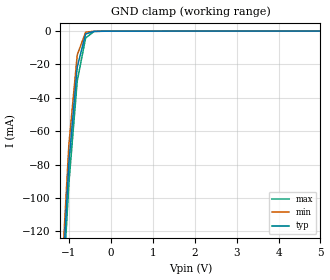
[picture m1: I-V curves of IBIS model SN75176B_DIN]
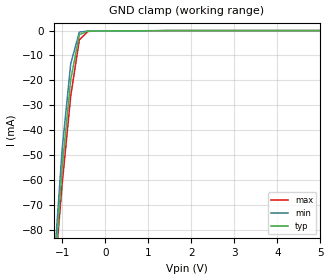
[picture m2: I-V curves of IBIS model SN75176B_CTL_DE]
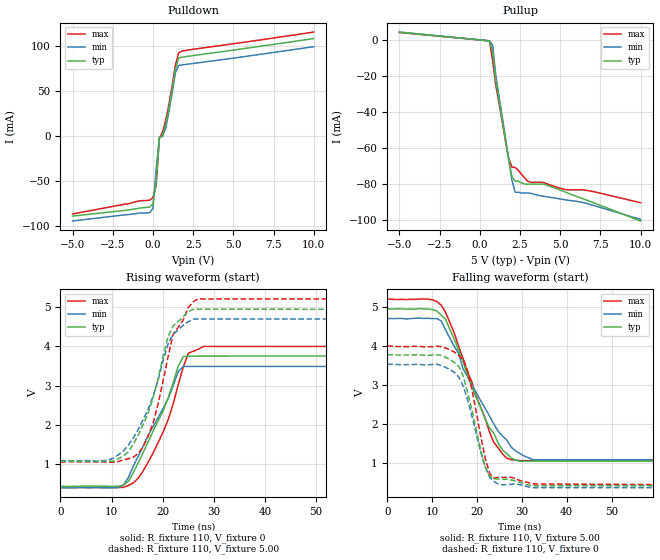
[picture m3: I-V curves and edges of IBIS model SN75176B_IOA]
|   TEXAS INSTRUMENTS INCORPORATED
|   Standard Linear and Logic Group
|   IBIS Model of SN75176
|   DIFFERENTIAL BUS TRANSCEIVERS
|   DIP 8-pin(P), SOL 8-pin(D), SOP 8-pin(PS)
[IBIS Ver]   3.1
[Comment char] |_char
[File Name]   sn75176b.ibs
[File Rev]   1.1
[Date]   Apr 26, 2004
[Source]   File originated at Texas Instruments, Inc
[Notes]   The following is a sample IBIS file for the SN75176B.
   - FILE REV HISTORY
   - 1.1 Release IBIS file on 04/29/04
   - All test data contained in this file are derived from
   actual measurement.
   - The measurement used P package.
   - We have data across voltage and temperature, but not across
   process.
[Disclaimer] Property of Texas Instruments Incorporated.  Unauthorized
   reproduction and/or distribution is strictly prohibited.
   This product is protected under copyright law.
   Created  2002, (C) Copyright  2002, Texas Instruments
   Incorporated, All Rights Reserved
   UNLESS THERE IS A SIGNED, WRITTEN AGREEMENT TO THE
   CONTRARY, TEXAS INSTRUMENTS (TI) IS PROVIDING THE IBIS
   MODELS  AND WITHOUT ANY WARRANTY, EXPRESSED OR
   IMPLIED.  TI assumes no liability for:
   1) the accuracy of the IBIS models provided to your
   company;
   2) the proper functioning of these IBIS Models in your
   design or for any resulting applications; or
   3) infringement of patents, copyrights or intellectual
   property rights resulting from your use of these IBIS
   models.
   TI provides IBIS Models as a service to our customers.
   You and your company shall not distribute, sell or give
   these models to anyone else without prior written
   permission from TI.
   TI reserves the right to make changes to our products or
   to discontinue any semiconductor product or service
   without notice, and advises our customers to obtain the
   latest version of relevant information to verify, before
   placing orders, that the information being relied on is
   current.
   Please be aware that your receipt and use of the IBIS
   information provided shall serve as acceptance of these
   terms and conditions.  If you do not accept these terms,
   you should return or destroy the IBIS models and any
   other accompanying information immediately.
|   Component SN75176B_P
[Component]   SN75176B_P
[Manufacturer]  Texas Instruments, Inc.
[Package]
|   typ   min   max
R_pkg   0.053   0.052   0.053
L_pkg   6.102nH   5.451nH   7.156nH
C_pkg   0.373pF   0.335pF   0.408pF
[Pin]   signal_name   model_name   R_pin   L_pin   C_pin
1   R   SN75176B_ROUT   0.052   7.146nH   0.387pF
2   RE_BAR   SN75176B_CTL_RE   0.053   5.451nH   0.408pF
3   DE   SN75176B_CTL_DE   0.053   5.513nH   0.370pF
4   D   SN75176B_DIN   0.053   6.304nH   0.336pF
5   GND   GND   0.052   6.295nH   0.335pF
6   A   SN75176B_IOA   0.053   5.499nH   0.356pF
7   B   SN75176B_IOB   0.053   5.452nH   0.404pF
8   VCC   POWER   0.053   7.156nH   0.387pF
|   Component  SN75176B_D
[Component]   SN75176B_D
[Manufacturer]  Texas Instruments, Inc.
[Package]
|   typ   min   max
R_pkg   0.026   0.017   0.035
L_pkg   2.637nH   2.180nH   3.093nH
C_pkg   0.269pF   0.224pF   0.313pF
[Pin]   signal_name   model_name   R_pin   L_pin   C_pin
1   R   SN75176B_ROUT   0.035   3.093nH   0.313pF
2   RE_BAR   SN75176B_CTL_RE   0.017   2.180nH   0.224pF
3   DE   SN75176B_CTL_DE   0.017   2.180nH   0.224pF
4   D   SN75176B_DIN   0.035   3.093nH   0.313pF
5   GND   GND   0.035   3.093nH   0.313pF
6   A   SN75176B_IOA   0.017   2.180nH   0.224pF
7   B   SN75176B_IOB   0.017   2.180nH   0.224pF
8   VCC   POWER   0.035   3.093nH   0.313pF
|   Component SN75176B_PS
[Component]   SN75176B_PS
[Manufacturer]  Texas Instruments, Inc.
[Package]
|   typ   min   max
R_pkg   0.031   0.030   0.032
L_pkg   2.946nH   2.774nH   3.117nH
C_pkg   0.201pF   0.154pF   0.248pF
[Pin]   signal_name   model_name   R_pin   L_pin   C_pin
1   R   SN75176B_ROUT   0.030   3.117nH   0.248pF
2   RE_BAR   SN75176B_CTL_RE   0.032   2.774nH   0.154pF
3   DE   SN75176B_CTL_DE   0.032   2.774nH   0.154pF
4   D   SN75176B_DIN   0.030   3.117nH   0.248pF
5   GND   GND   0.030   3.117nH   0.248pF
6   A   SN75176B_IOA   0.032   2.774nH   0.154pF
7   B   SN75176B_IOB   0.032   2.774nH   0.154pF
8   VCC   POWER   0.030   3.117nH   0.248pF
| Models and submodels in the file (6): SN75176B_DIN (Input), SN75176B_CTL_DE (Input), SN75176B_IOA (I/O), SN75176B_IOB (I/O), SN75176B_CTL_RE (Input), SN75176B_ROUT (Output)
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|   Model SN75176B_DIN
[Model]   SN75176B_DIN
Model_type  Input
Polarity   Non-Inverting
Vinl = 0.8
Vinh = 2.0
| variable   typ   min   max
C_comp   3.886pf   3.848pf   3.932pf
[Temperature Range]   40   0   85
| Ambient temperature   25   0   70
[Voltage Range]   5.00   4.75   5.25
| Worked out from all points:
|   GND clamp passes 1 mA (typ) near -0.51 V on its own axis
[GND Clamp]
|   Voltage   I(typ)   I(min)   I(max)
-5V       -2.345A    -2.465A    -2.196A
-1.2V     -170.8mA   -160.5mA   -180.4mA
-1V       -79.55mA   -68.35mA   -91.64mA
-800mV    -21.57mA   -14.32mA   -29.9mA
-600mV    -1.753mA   -653.7uA   -4.151mA
-400mV    -130.2uA   -114uA     -258.2uA
-200mV    -95.23uA   -90.83uA   -97.44uA
5V        442.5pA    263.9pA    1.111nA
|   Model SN75176B_CTL_DE
[Model]   SN75176B_CTL_DE
Model_type  Input
Polarity   Non-Inverting
Vinl = 0.8
Vinh = 2.0
| variable   typ   min   max
C_comp   3.080pf   3.073pf   3.123pf
[Temperature Range]   40   0   85
| Ambient temperature   25   0   70
[Voltage Range]   5.00   4.75   5.25
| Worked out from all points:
|   GND clamp passes 1 mA (typ) near -0.51 V on its own axis
[GND Clamp]
|   Voltage   I(typ)   I(min)   I(max)
-5V       -1.071A    -1.14A     -1.043A
-1.2V     -104.3mA   -97.42mA   -103.9mA
-1V       -55.02mA   -47.73mA   -61.82mA
-800mV    -19.7mA    -13.26mA   -26.25mA
-600mV    -1.618mA   -611.8uA   -3.698mA
-400mV    -217.2uA   -198.8uA   -322.9uA
-200mV    -174.5uA   -165.2uA   -179.4uA
5V        105.1pA    41.86pA    432.2pA
|   Model SN75176B_IOA
[Model]   SN75176B_IOA
Model_type  I/O
Polarity   Non-Inverting
Enable   Active-High
Vinl = 2.2
Vinh = 2.8
| variable   typ   min   max
C_comp   14.112pf   12.360pf   14.223pf
[Temperature Range]   40   0   85
| Ambient temperature   25   0   70
[Voltage Range]   5.00   4.75   5.25
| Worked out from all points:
|   slope of the pulldown table from 0 to 0.75 V, typ, clamps not added: 8.73 ohm
|   slope of the pullup table from 0 to 0.75 V, typ, clamps not added: 140 ohm
|   rising waveform, R_fixture 110, V_fixture 0: 20-80 % time 6.63ns typ, 7.14ns min, 6.14ns max; typ from 0.43 V to 3.75 V
|   falling waveform, R_fixture 110, V_fixture 5.00: 20-80 % time 8.34ns typ, 9.77ns min, 7.77ns max; typ from 4.95 V to 1.05 V
|   rising waveform, R_fixture 110, V_fixture 5.00: 20-80 % time 5.31ns typ, 5.99ns min, 4.74ns max; typ from 1.07 V to 4.95 V
|   falling waveform, R_fixture 110, V_fixture 0: 20-80 % time 4.19ns typ, 4.42ns min, 3.72ns max; typ from 3.78 V to 0.423 V
[Pulldown]
|   Voltage   I(typ)   I(min)   I(max)
-5V       -88.68mA   -94.13mA   -86.33mA
-200mV    -78.65mA   -84.9mA    -70.92mA
0V        -75.16mA   -80.07mA   -68.17mA
200mV     -50.16mA   -36.86mA   -54.7mA
400mV     -1.786mA   -960.3uA   -2.31mA
600mV     1.463mA    -130.5uA   4.87mA
800mV     13.8mA     9.488mA    18.53mA
1V        31.84mA    27.92mA    36.08mA
1.4V      75.01mA    70.88mA    79.19mA
1.6V      87.06mA    78.84mA    92.77mA
2V        88.55mA    79.88mA    95.48mA
10V       108.8mA    99.68mA    116mA
[Pullup]
|   Voltage   I(typ)   I(min)   I(max)
-5V       4.497mA    4.59mA     4.307mA
600mV     -323.8uA   -325uA     -422.5uA
800mV     -6.738mA   -2.755mA   -11.39mA
1V        -22.79mA   -19.92mA   -25.11mA
1.8V      -66.71mA   -66.15mA   -65.79mA
2V        -75.74mA   -77.68mA   -70.41mA
2.2V      -78.17mA   -84.34mA   -70.57mA
3V        -79.82mA   -84.74mA   -78.32mA
4V        -79.82mA   -86.64mA   -79.04mA
5.4V      -84.55mA   -88.64mA   -82.98mA
6.4V      -87.91mA   -90mA      -82.98mA
10V       -100.3mA   -99.39mA   -90.17mA
[Ramp]
| variable   typ   min   max
dV/dt_r  2.04E+00/6.70E-09  2.07E+00/7.70E-09  2.20E+00/6.20E-09
dV/dt_f  2.06E+00/4.30E-09  2.04E+00/4.80E-09  2.05E+00/3.61E-09
R_load = 110
[Rising Waveform]
R_fixture = 110
V_fixture = 0
V_fixture_min = 0
V_fixture_max = 0
C_fixture = 0pf
L_fixture = 0nH
|   Time   V(typ)   V(min)   V(max)
0s        430.5mV    393.5mV    400.5mV
11.15ns   429.8mV    395.8mV    400.4mV
12.32ns   458.1mV    463.1mV    404.6mV
14.27ns   778.8mV    947.7mV    517.6mV
20.13ns   2.369V     2.426V     1.831V
23.06ns   3.503V     3.362V     3.034V
24.04ns   3.739V     3.487V     3.48V
25.02ns   3.748V     3.487V     3.824V
27.97ns   3.75V      3.487V     3.996V
75.2ns    3.75V      3.487V     3.996V
[Falling Waveform]
R_fixture = 110
V_fixture = 5.00
V_fixture_min = 4.75
V_fixture_max = 5.25
C_fixture = 0pf
L_fixture = 0nH
|   Time   V(typ)   V(min)   V(max)
0s        4.951V     4.703V     5.203V
10.06ns   4.933V     4.701V     5.182V
12.02ns   4.788V     4.642V     5.046V
15.05ns   4.146V     3.968V     4.295V
19.83ns   2.68V      2.803V     2.705V
23.73ns   1.772V     2.007V     1.535V
26.66ns   1.245V     1.591V     1.125V
28.62ns   1.081V     1.312V     1.076V
32.52ns   1.054V     1.086V     1.066V
75.2ns    1.054V     1.089V     1.066V
[Rising Waveform]
R_fixture = 110
V_fixture = 5.00
V_fixture_min = 4.75
V_fixture_max = 5.25
C_fixture = 0pf
L_fixture = 0nH
|   Time   V(typ)   V(min)   V(max)
0s        1.066V     1.074V     1.049V
10.3ns    1.077V     1.149V     1.044V
13.23ns   1.305V     1.473V     1.133V
15.18ns   1.722V     1.872V     1.266V
18.11ns   2.685V     2.724V     2.042V
21.04ns   4.239V     4.057V     3.723V
22.02ns   4.515V     4.299V     4.304V
24.97ns   4.883V     4.622V     4.981V
26.92ns   4.945V     4.696V     5.208V
75.2ns    4.947V     4.689V     5.2V
[Falling Waveform]
R_fixture = 110
V_fixture = 0
V_fixture_min = 0
V_fixture_max = 0
C_fixture = 0pf
L_fixture = 0nH
|   Time   V(typ)   V(min)   V(max)
0s        3.778V     3.532V     4.003V
12.11ns   3.756V     3.496V     3.981V
16.02ns   3.466V     3.195V     3.75V
16.99ns   3.206V     2.957V     3.635V
18.95ns   2.32V      2.17V      2.84V
21.88ns   895.1mV    884.4mV    1.108V
22.85ns   667.7mV    640mV      728.5mV
23.83ns   602.9mV    528.7mV    621.2mV
32.62ns   423.5mV    372.7mV    471mV
75.2ns    423.3mV    370.9mV    445.7mV
